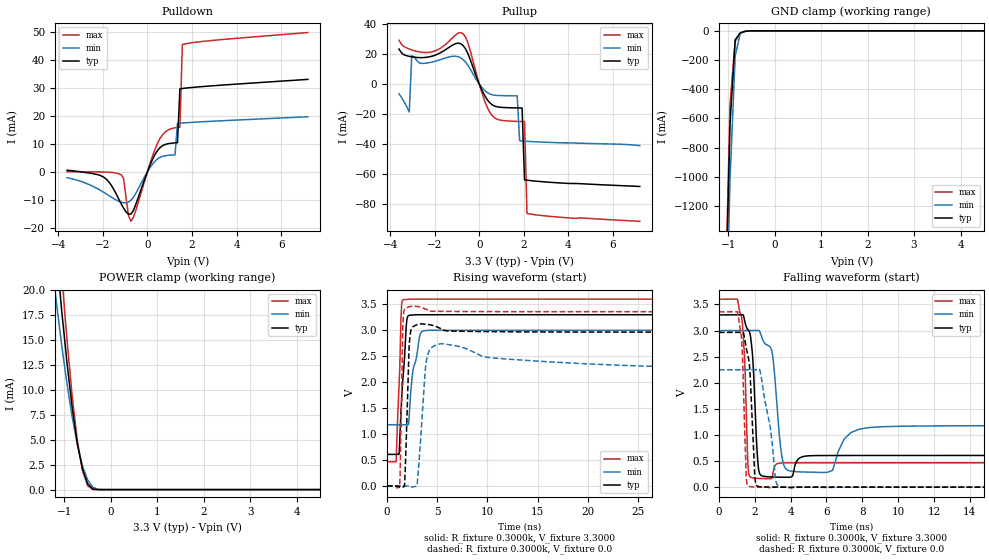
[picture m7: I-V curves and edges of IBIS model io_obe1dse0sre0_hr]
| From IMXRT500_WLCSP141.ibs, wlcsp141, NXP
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[Model] io_obe1dse0sre0_hr
|   Model io_obe1dse0sre0_hr
| Library cells for typ/min/max conditions are connected as defined below:
|  pad - External Pad
|  ipp_do - Core Input
|  ipp_obe - Output Buffer Enable
|  REFH3V3 - vdd1v8
|  REFL3V3 - vdd1v8
|  gnde - gnde
|  ipp_ina235_3v - NC
|  ipp_ina40_3v - NC
|  ipp_ina_mux - NC
|  ipp_ind - NC
|  ipp_ind_1p8v - NC
|  ipp_ind_3v - NC
|  vdd - vdd
|  vdd1v8 - vdd1v8
|  vdda - vdde3v3
|  vdde3v3 - vdde3v3
| All other pins connected to ground
Model_type I/O
Polarity   Non-Inverting
Enable   Active-High
Vinl =   0.9900V
Vinh =   2.3100V
Vmeas =  1.6500V
Cref =   25.0000pF
Rref =   0.5000k
Vref =   0.0V
C_comp   1.8292pF   1.7593pF   1.9120pF
[Temperature Range]   25.0000   0.1250k   -40.0000
[Voltage Range]   3.3000V   3.0000V   3.6000V
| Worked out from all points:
|   slope of the pulldown table from 0 to 0.495 V, typ, clamps not added: 61.4 ohm
|   slope of the pullup table from 0 to 0.495 V, typ, clamps not added: 38.6 ohm
|   GND clamp passes 1 mA (typ) near -0.55 V on its own axis
|   POWER clamp passes 1 mA (typ) near -0.53 V on its own axis
|   rising waveform, R_fixture 0.3000k, V_fixture 3.3000: 20-80 % time 489ps typ, 789ps min, 328ps max; typ from 0.608 V to 3.3 V
|   rising waveform, R_fixture 0.3000k, V_fixture 0.0: 20-80 % time 277ps typ, 468ps min, 177ps max; typ from 0 V to 2.96 V
|   falling waveform, R_fixture 0.3000k, V_fixture 3.3000: 20-80 % time 254ps typ, 312ps min, 208ps max; typ from 3.3 V to 0.608 V
|   falling waveform, R_fixture 0.3000k, V_fixture 0.0: 20-80 % time 254ps typ, 572ps min, 185ps max; typ from 2.96 V to 0 V
[Pulldown]
|Voltage   I(typ)   I(min)   I(max)
-3.6V     580uA      -2.07mA    30uA
-1.95V    -1.94mA    -7.35mA    -60uA
-1.18V    -11.35mA   -10.84mA   -1.013mA
-1.07V    -12.94mA   -11.04mA   -2.193mA
-850mV    -15.13mA   -10.79mA   -15.56mA
-740mV    -15.14mA   -10.18mA   -17.69mA
470mV     7.826mA    4.727mA    10.49mA
1.24V     10.39mA    6.092mA    15.78mA
1.35V     10.45mA    17.36mA    15.91mA
1.46V     29.75mA    17.44mA    16.02mA
1.57V     29.87mA    17.51mA    45.62mA
7.2V      33.13mA    19.73mA    49.89mA
[Pullup]
|Voltage   I(typ)   I(min)   I(max)
-3.6V     23.39mA    -6.412mA   29.31mA
-3.14V    18.55mA    -18.52mA   23.46mA
-3.03V    18.24mA    18.95mA    22.87mA
-2.04V    19.01mA    15.03mA    21.91mA
-720mV    25.7mA     16.34mA    33.57mA
490mV     -12.7mA    -6.677mA   -19.19mA
1.7V      -15.88mA   -7.809mA   -24.84mA
1.81V     -15.91mA   -37.73mA   -24.9mA
1.92V     -15.95mA   -37.88mA   -24.96mA
2.03V     -63.83mA   -38.01mA   -25.02mA
2.14V     -64.06mA   -38.13mA   -86.3mA
7.2V      -68.26mA   -41.02mA   -91.5mA
[GND_clamp]
|Voltage   I(typ)   I(min)   I(max)
-3.6V     -46.64A    -46.27A    -48.09A
-1.07V    -2.038A    -2.424A    -1.965A
-960mV    -629.9mA   -1.012A    -499.2mA
-850mV    -61.62mA   -174.1mA   -72.03mA
-740mV    -13.6mA    -15.66mA   -16.3mA
-630mV    -2.66mA    -3.244mA   -3.912mA
-410mV    -9.358uA   -49.22uA   -3.515uA
7.2V      0A         0A         0A
[POWER_clamp]
|Voltage   I(typ)   I(min)   I(max)
-3.6V     129.4mA    109.3mA    143.3mA
-1.27V    28.99mA    22.71mA    35.27mA
-1.16V    23.09mA    18.31mA    28mA
-1.05V    17.57mA    14.21mA    21.12mA
-940mV    12.56mA    10.49mA    14.82mA
-830mV    8.174mA    7.224mA    9.263mA
-720mV    4.592mA    4.483mA    4.857mA
-610mV    2.058mA    2.37mA     1.909mA
-500mV    597.2uA    970.5uA    391.6uA
-390mV    63.24uA    245.6uA    14.23uA
-170mV    54.62nA    1.775uA    12.62nA
7.2V      0A         0A         0A
[Ramp]
| variable   typ   min   max
dV/dt_r  0.6639/0.3114n   0.7715/1.4878n   0.7549/0.1573n
dV/dt_f  0.9021/0.3658n   0.5338/0.4070n   1.3523/0.3211n
R_load = 50.0000
[Rising Waveform]
R_fixture= 0.3000k
V_fixture= 3.3000
V_fixture_min= 3.0000
V_fixture_max= 3.6000
|time   V(typ)   V(min)   V(max)
0s        607.6mV    1.179V     467.4mV
902.6ps   607.6mV    1.179V     473.4mV
1.204ns   622.5mV    1.179V     1.941V
1.467ns   1.708V     1.179V     3.513V
1.934ns   3.127V     1.179V     3.594V
2.184ns   3.288V     1.274V     3.6V
2.541ns   3.294V     2.167V     3.601V
3.238ns   3.3V       2.871V     3.6V
4.163ns   3.3V       3V         3.6V
500ns     3.3V       3V         3.6V
[Rising Waveform]
R_fixture= 0.3000k
V_fixture= 0.0
V_fixture_min= 0.0
V_fixture_max= 0.0
|time   V(typ)   V(min)   V(max)
0s        327.7nV    1.778uV    1.402uV
1.259ns   -25.44mV   1.744uV    -6.504mV
1.558ns   -21.48mV   1.517uV    2.977V
1.732ns   -2.424mV   1.198uV    3.4V
2.2ns     2.668V     -18.63mV   3.454V
2.53ns    3.061V     -19.13mV   3.466V
3.029ns   3.109V     86.28mV    3.458V
3.932ns   3.116V     2.426V     3.4V
5.364ns   3.03V      2.742V     3.365V
500ns     2.965V     2.248V     3.358V
[Falling Waveform]
R_fixture= 0.3000k
V_fixture= 3.3000
V_fixture_min= 3.0000
V_fixture_max= 3.6000
|time   V(typ)   V(min)   V(max)
0s        3.3V       3V         3.6V
1.276ns   3.299V     3V         3.237V
1.715ns   2.965V     3V         209.8mV
2.207ns   359.6mV    3.002V     167.7mV
2.772ns   198.7mV    2.71V      161.9mV
3.644ns   190mV      403.2mV    465.7mV
5.82ns    606.5mV    281.9mV    467.4mV
7.39ns    607.4mV    1.051V     467.4mV
12.3ns    607.7mV    1.175V     467.4mV
500ns     607.6mV    1.179V     467.4mV
[Falling Waveform]
R_fixture= 0.3000k
V_fixture= 0.0
V_fixture_min= 0.0
V_fixture_max= 0.0
|time   V(typ)   V(min)   V(max)
0s        2.965V     2.248V     3.358V
1.058ns   2.965V     2.248V     3.331V
1.288ns   2.967V     2.248V     2.726V
1.575ns   2.585V     2.248V     53.83mV
1.733ns   2.204V     2.248V     11.5mV
2.044ns   89.46mV    2.249V     3.619mV
2.92ns    2.278mV    997mV      -12.88mV
3.285ns   1.624mV    34.31mV    855.3uV
5.936ns   374.8uV    -5.22mV    27.79uV
500ns     1.533uV    3.286uV    3.233uV
